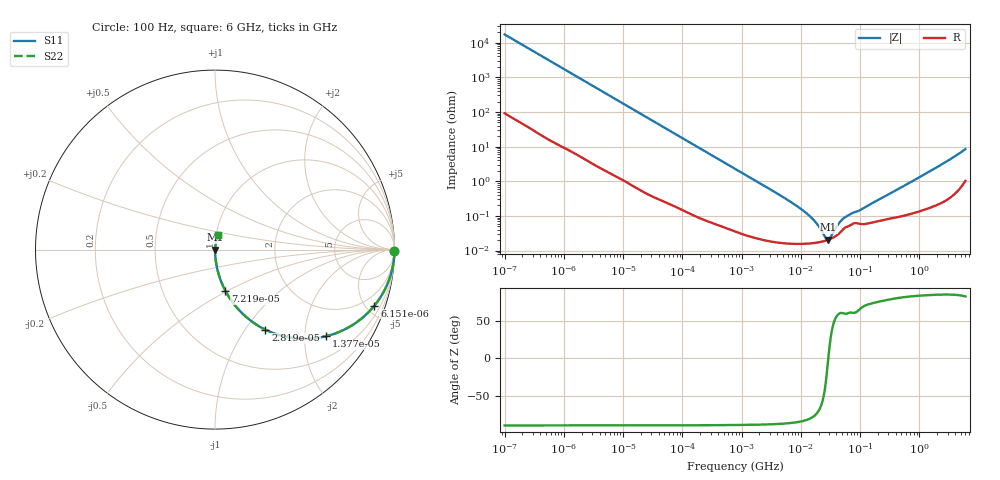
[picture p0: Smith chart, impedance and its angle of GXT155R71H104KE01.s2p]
!Murata Part Number: GXT155R71H104KE01
!These Parameters are Measured in Series Mode Connection
!Data Generated on Jan 08, 2026
!  o--ll--o
!Port1  Port2
!  o------o
!Operation Temp=25[degC], DC Bias Voltage=0[V]
!Freq. Start=100[Hz] Stop=6[GHz] 401[Steps]
# Hz S RI R 50
!Freq.(Hz) S11(Real) S11(Imag) S21(Real) S21(Imag) S12(Real) S12(Imag) S22(Real) S22(Imag)
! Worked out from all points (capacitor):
!   401 points, 100 Hz to 6 GHz, reference 50 ohm
!   read as one part in series: C = 92.2 nF near 109 Hz
!   lowest |Z| = 20.5 mohm at 29.12 MHz (marker M1)
!   series resonance near 29.1 MHz, so ESL is about 320 pH
!   S11 on the Smith chart (normalised r, x): 100 Hz: open; 6.151 kHz: 1.03, -5.68; 13.77 kHz: 1.02, -2.55; 28.19 kHz: 1.01, -1.25; 72.19 kHz: 1.00, -0.49; 6 GHz: 1.02, +0.17
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100  0.9999 -0.0058  6.44e-05 0.0058  6.44e-05 0.0058  0.9999 -0.0058
627  0.9985 -0.0361  0.00149 0.0361  0.00149 0.0361  0.9985 -0.0361
2008  0.9862 -0.1137  0.0138 0.1137  0.0138 0.1137  0.9862 -0.1137
6151  0.8883 -0.312  0.1117 0.312  0.1117 0.312  0.8883 -0.312
9204  0.782 -0.4099  0.218 0.4099  0.218 0.4099  0.782 -0.4099
13772  0.6177 -0.4829  0.3823 0.4829  0.3823 0.4829  0.6177 -0.4829
19704  0.4428 -0.4937  0.5572 0.4937  0.5572 0.4937  0.4428 -0.4937
28191  0.2811 -0.4464  0.7189 0.4464  0.7189 0.4464  0.2811 -0.4464
40335  0.1616 -0.3647  0.8384 0.3647  0.8384 0.3647  0.1616 -0.3647
72189  0.058 -0.2298  0.942 0.2298  0.942 0.2298  0.058 -0.2298
193316  0.00919 -0.0908  0.9908 0.0908  0.9908 0.0908  0.00919 -0.0908
774597  0.000886 -0.023  0.9991 0.023  0.9991 0.023  0.000886 -0.023
6644369  0.000164 -0.00258  0.9998 0.00258  0.9998 0.00258  0.000164 -0.00258
1.555665e7  0.000163 -0.00083  0.9998 0.00083  0.9998 0.00083  0.000163 -0.00083
1.946e7  0.000172 -0.000514  0.9998 0.000514  0.9998 0.000514  0.000172 -0.000514
2.662322e7  0.000195 -0.000111  0.9998 0.000111  0.9998 0.000111  0.000195 -0.000111
2.911731e7  0.000205 7e-07  0.9998 -7e-07  0.9998 -7e-07  0.000205 7e-07
3.184506e7  0.000218 0.000112  0.9998 -0.000112  0.9998 -0.000112  0.000218 0.000112
4.35672e7  0.000303 0.000515  0.9997 -0.000515  0.9997 -0.000515  0.000303 0.000515
5.449875e7  0.000445 0.00077  0.9996 -0.00077  0.9996 -0.00077  0.000445 0.00077
3.124326e8  0.000844 0.00424  0.9992 -0.00424  0.9992 -0.00424  0.000844 0.00424
6e9  0.017 0.0819  0.983 -0.0819  0.983 -0.0819  0.017 0.0819
